PROGRAM KITCHEN
VAR	
	fbLight1: FB_Light;
	fbLight2: FB_Light;
	fbLight3: FB_Light;
	
	R_TRIG_BlindUp: R_TRIG;	
	R_TRIG_BlindDown: R_TRIG;
	bSwitchBlindUp: BOOL;
	bSwitchBlindDown: BOOL;
	fbVenetianBlind: FB_VenetianBlind;	
END_VAR

// Light 1
fbLight1(bOn:= , bOff:= , bToggle:= GVL.I_bTerm1_Var1, bLight=> GVL.Q_bTerm3_Var1);

// Light 2
fbLight2(bOn:= , bOff:= , bToggle:= GVL.I_bTerm1_Var2, bLight=> GVL.Q_bTerm3_Var2);
	
// Light 3
fbLight3(bOn:= , bOff:= , bToggle:= GVL.I_bTerm1_Var3, bLight=> GVL.Q_bTerm3_Var3);
	
// Blind 1
R_TRIG_BlindUp(CLK:=GVL.I_bTerm1_Var4);
bSwitchBlindUp:=R_TRIG_BlindUp.Q;
R_TRIG_BlindDown(CLK:=GVL.I_bTerm1_Var5);
bSwitchBlindDown:= R_TRIG_BlindDown.Q;

fbVenetianBlind(
	bUp:= bSwitchBlindUp, 
	bDown:= bSwitchBlindDown, 
	bStop:= (bSwitchBlindUp OR bSwitchBlindDown) AND (fbVenetianBlind.bBlindUp OR fbVenetianBlind.bBlindDown), 
	bSwitchOverUp:= , 
	bSwitchOverDown:= , 
	tSwitchOverTime:= , 
	bStepUp:= , 
	bStepDown:= , 
	tStepTime:= , 
	bShadowPosition:= , 
	tShadowTurnAroundTime:= , 
	tShadowTurnOffTime:= , 
	bSafetyPosition:= , 
	tTurnOffTime:= , 
	tSwitchOverDeadTime:= , 
	bBlindUp=> GVL.Q_bTerm6_Var1, 
	bBlindDown=> GVL.Q_bTerm6_Var2);

END_PROGRAM
